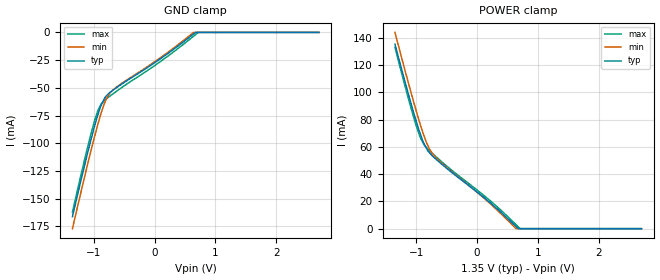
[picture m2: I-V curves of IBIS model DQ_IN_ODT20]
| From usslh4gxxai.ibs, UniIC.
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| MODEL DQ_IN_ODT20 (Data Input with 20ohm ODT, 800-2133Mbps)
[Model]   DQ_IN_ODT20
Model_type   Input
Vinl = 545.000mV
Vinh = 805.000mV
|   typ   min   max
|C_comp   1.035pF   0.986pF   1.103pF
C_comp_power_clamp   0.5175pF   0.4930pF   0.5515pF
C_comp_gnd_clamp   0.5175pF   0.4930pF   0.5515pF
| Note: C_comp changes when the ODT circuit is enabled.
[Model Spec]
| Input threshold voltage corners
Vinl   0.5450V   0.5115V   0.5825V
Vinh   0.8050V   0.7715V   0.8425V
| Dynamic Overshoot Parameters from DDR3L Specification
|D_overshoot_ampl_h   0.40   NA   NA
|D_overshoot_ampl_l   0.40   NA   NA
|D_overshoot_area_h   0.11n   NA   NA
|D_overshoot_area_l   0.11n   NA   NA
[Receiver Thresholds]
Vth   =  0.675V
Vth_min  =  0.6615V
Vth_max  =  0.6885V
Vinh_ac  =  0.130V
Vinh_dc  =  0.090V
Vinl_ac  = -0.130V
Vinl_dc  = -0.090V
Tslew_ac =  5.000ns |Not specified, so set to high value
Threshold_sensitivity = 0.50
Reference_supply Power_clamp_ref
[Voltage Range]   1.3500V   1.2830V   1.4250V
[POWER Clamp Reference]   1.3500V   1.2830V   1.4250V
[Temperature Range]   45.0   95.0   -40.0
[GND Clamp]
|   Voltage   I(typ)   I(min)   I(max)
-1.35V    -166.3mA   -177.1mA   -162.2mA
-1.11V    -110.8mA   -121mA     -105.5mA
-990mV    -85.35mA   -94.61mA   -80.22mA
-935mV    -74.97mA   -83.31mA   -70.92mA
-885mV    -66.4mA    -73.78mA   -65.36mA
-810mV    -58.2mA    -62.2mA    -60.6mA
-785mV    -56.84mA   -58.97mA   -59.54mA
-680mV    -51.97mA   -51.62mA   -55.27mA
110mV     -23.21mA   -22.26mA   -25.7mA
640mV     -1.463mA   0A         -3.434mA
718mV     0A         0A         0A
2.7V      0A         0A         0A
[POWER Clamp]
|   Voltage   I(typ)   I(min)   I(max)
-1.35V    135.5mA    144.1mA    133.2mA
-1.11V    95.68mA    103.8mA    92.36mA
-990mV    77.3mA     84.75mA    74mA
-930mV    69.11mA    75.86mA    66.49mA
-885mV    63.46mA    69.61mA    62.66mA
-780mV    55.58mA    58.21mA    57.08mA
-730mV    53.18mA    54.8mA     55.01mA
-590mV    47.64mA    48.4mA     49.42mA
115mV     22.74mA    22.32mA    24.22mA
640mV     1.535mA    94.48uA    2.93mA
707mV     0A         0A         0A
2.7V      0A         0A         0A
